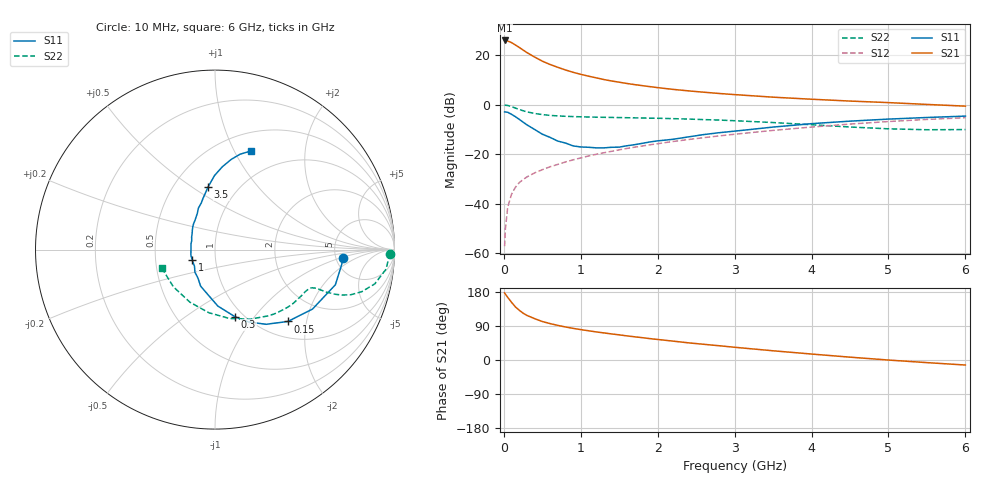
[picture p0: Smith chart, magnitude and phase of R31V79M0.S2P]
! SIEMENS Small Signal Semiconductors
! BFR181
! Si NPN RF Bipolar Junction Transistor in SOT23
! VCE = 1.75 V  IC = 9 mA
! Common Emitter S-Parameters:  May  1996
# GHz  S  MA  R  50
!  f  S11  S21  S12  S22
! GHz  MAG  ANG  MAG  ANG  MAG  ANG  MAG  ANG
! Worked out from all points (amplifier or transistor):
!   36 points, 10 MHz to 6 GHz, reference 50 ohm
!   highest |S21| = 25.8 dB at 10 MHz (marker M1)
!   |S21| within 3 dB of that: start of sweep to 209.2 MHz
!   unconditionally stable (mu >= 1): 674.5 MHz to 2.759 GHz
!   at 250 MHz: K = 0.62, MSG = 26.1 dB, |S12| = -30.2 dB
!   at 1.4 GHz: K = 1.10, MAG = 12.3 dB, |S12| = -18.8 dB
!   at 6 GHz: K = 0.87, MSG = 2.3 dB, |S12| = -5.3 dB
!   S11 on the Smith chart (normalised r, x): 10 MHz: 5.76, -1.05; 150 MHz: 1.32, -1.56; 300 MHz: 0.91, -0.81; 1 GHz: 0.77, -0.09; 3.5 GHz: 0.73, +0.58; 6 GHz: 0.70, +1.17
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0.01  0.7127 -3.6  19.61 177.0  0.0014 84.0  0.9767 -1.3
0.02  0.7109 -6.7  19.46 173.8  0.0031 84.3  0.9699 -2.6
0.05  0.6987 -16.3  19.09 165.4  0.0085 81.1  0.9593 -6.5
0.1  0.6362 -31.4  17.74 152.2  0.0156 76.8  0.9107 -12.1
0.15  0.5702 -44.6  15.91 140.2  0.0215 71.0  0.8506 -16.0
0.2  0.5043 -55.6  14.19 131.3  0.0267 68.2  0.7972 -18.4
0.25  0.4433 -65.3  12.58 123.6  0.0308 66.0  0.7509 -19.7
0.3  0.3904 -73.4  11.18 117.7  0.0348 66.0  0.7137 -20.4
0.4  0.3151 -87.1  9.085 109.1  0.042 65.9  0.6624 -20.9
0.5  0.253 -99.2  7.508 101.6  0.0487 66.8  0.6286 -20.9
0.6  0.2187 -111.5  6.441 96.1  0.0557 67.3  0.6055 -20.9
0.7  0.1841 -121.2  5.645 91.4  0.0622 68.2  0.5911 -21.2
0.8  0.1681 -131.8  4.991 87.2  0.0696 68.3  0.5808 -21.5
1  0.1398 -155.2  4.07 80.2  0.084 69.2  0.5673 -22.7
1.1  0.1379 -166.7  3.743 77.2  0.0921 69.2  0.5619 -23.5
1.3  0.134 175.2  3.199 71.5  0.1069 69.2  0.5534 -25.3
1.6  0.148 151.6  2.662 63.6  0.1305 68.4  0.5437 -28.8
2.2  0.1997 123.5  2.025 49.8  0.1804 65.5  0.5207 -37.2
3.5  0.3521 96.2  1.41 24.3  0.3016 55.0  0.4344 -63.2
4.5  0.4636 84.9  1.177 7.5  0.4045 43.4  0.3532 -95.7
5.5  0.5494 75.3  1.007 -6.9  0.502 29.9  0.3111 -138.1
6  0.5855 69.9  0.93 -13.3  0.5448 22.5  0.3135 -160.5
